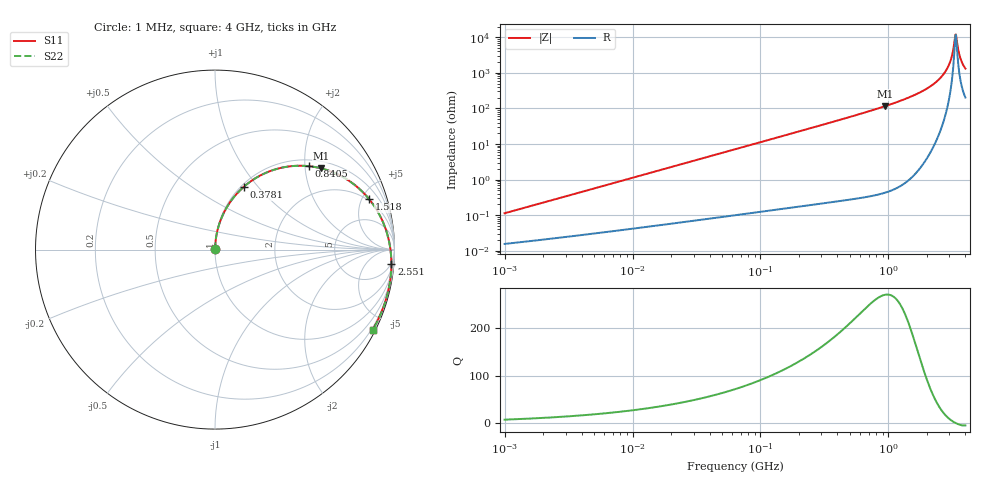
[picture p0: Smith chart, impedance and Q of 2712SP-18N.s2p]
# MHz  S  MA  R  50
!Freq  MagS11  AngS11  MagS21  AngS21  MagS12  AngS12  MagS22  AngS22
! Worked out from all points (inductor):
!   801 points, 1 MHz to 4 GHz, reference 50 ohm
!   read as one part in series: L = 17.9 nH near 1.042 MHz
!   highest Q = 270 at 942.1 MHz (marker M1), where L = 19.6 nH
!   self-resonance near 3.341 GHz
!   S11 on the Smith chart (normalised r, x): 1 MHz: 1.00, +0.00; 378.1 MHz: 1.03, +0.84; 840.5 MHz: 1.15, +2.10; 1.518 GHz: 1.85, +5.70; 2.551 GHz: 4, -24; 4 GHz: 0.13, -4.15
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1  0.001097 81.8  0.9998 -0.1  0.9998 -0.1  0.001097 81.8
4.016383  0.00437 86.1  0.9997 -0.3  0.9997 -0.3  0.00437 86.1
15.96482  0.01734 87.2  0.9993 -1.1  0.9993 -1.1  0.01734 87.2
63.45894  0.06873 84.9  0.9966 -4.2  0.9966 -4.2  0.06872 84.9
252.2445  0.2654 73.1  0.9623 -16.5  0.9623 -16.5  0.2653 73.1
378.0635  0.3839 65.4  0.9212 -24.2  0.9212 -24.2  0.3838 65.4
555.003  0.5273 55.5  0.8473 -34.3  0.8473 -34.3  0.5271 55.5
840.5134  0.6997 41.6  0.7118 -48.1  0.7118 -48.1  0.6994 41.6
942.1351  0.7457 37.4  0.6636 -52.4  0.6636 -52.4  0.7454 37.4
1013.11  0.7738 34.6  0.6307 -55.2  0.6307 -55.2  0.7734 34.6
1518.448  0.9041 18.1  0.4229 -71.6  0.4229 -71.6  0.9037 18.1
2051.543  0.9636 5.2  0.2559 -84.1  0.2559 -84.1  0.9633 5.2
2551.006  0.9858 -4.5  0.1373 -92.6  0.1373 -92.6  0.9858 -4.5
2800.706  0.9903 -8.9  0.08865 -95.3  0.08865 -95.3  0.9905 -8.9
2980.609  0.9918 -11.8  0.05746 -95.6  0.05746 -95.6  0.9921 -11.8
3106.919  0.9922 -13.8  0.03745 -93.5  0.03745 -93.5  0.9925 -13.8
3272.36  0.9919 -16.4  0.01439 -75.4  0.01439 -75.4  0.9925 -16.4
3340.977  0.9916 -17.4  0.008208 -37.5  0.008208 -37.5  0.9923 -17.4
3446.61  0.991 -19.0  0.01378 34.6  0.01378 34.6  0.9918 -19.0
3630.14  0.9895 -21.7  0.0344 53.1  0.0344 53.1  0.9905 -21.7
3744.916  0.9883 -23.4  0.0467 54.8  0.0467 54.8  0.9895 -23.4
4000  0.9854 -27.0  0.0708 54.2  0.0708 54.2  0.987 -27.1
